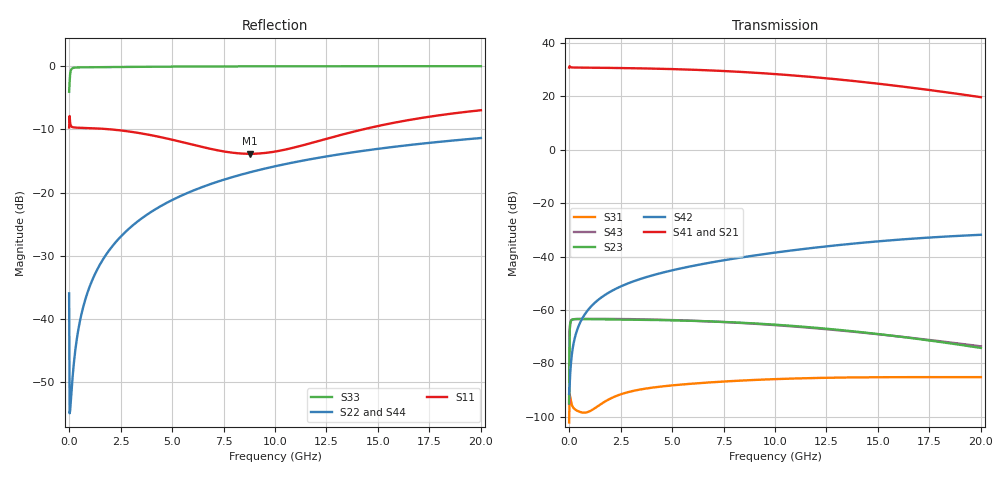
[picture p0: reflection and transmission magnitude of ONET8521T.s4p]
! *  ONET8521T
! * (C) Copyright 2011 Texas Instruments Incorporated. All rights reserved.
! ** This model is designed as an aid for customers of Texas Instruments.
! ** TI and its licensors and suppliers make no warranties, either expressed
! ** or implied, with respect to this model, including the warranties of
! ** merchantability or fitness for a particular purpose.  The model is
! ** provided solely on an "as is" basis.  The entire risk as to its quality
! ** and performance is with the customer.
! ** 1) THE ACCURACY OF THE MODELS PROVIDED TO YOUR COMPANY;
! ** 2) THE PROPER FUNCTIONING OF THESE MODELS IN YOUR DESIGN OR FOR ANY RESULTING
! ** APPLICATIONS; OR 3) INFRINGEMENT OF PATENTS, COPYRIGHTS OR INTELLECTUAL PROPERTY
! **  RIGHTS RESULTING FROM YOUR USE OF THESE HSPICE MODELS.
! ** TI PROVIDES MODELS AS A SERVICE TO OUR CUSTOMERS. YOU AND YOUR COMPANY
! ** SHALL NOT DISTRIBUTE, SELL OR GIVE THESE MODELS
! ** TO ANYONE ELSE WITHOUT PRIOR WRITTEN PERMISSION FROM TI.
! ** TI RESERVES THE RIGHT TO MAKE CHANGES TO OUR PRODUCTS OR TO DISCONTINUE
! ** ANY SEMICONDUCTOR PRODUCT OR SERVICE WITHOUT NOTICE, AND ADVISES OUR
! ** CUSTOMERS TO OBTAIN THE LATEST VERSION OF RELEVANT INFORMATION TO VERIFY,
! ** BEFORE PLACING ORDERS, THAT THE INFORMATION BEING RELIED ON IS CURRENT.
! ** PLEASE BE AWARE THAT YOUR RECEIPT AND USE OF THIS INFORMATION PROVIDED SHALL
! ** SERVE AS ACCEPTANCE OF THESE TERMS AND CONDITIONS. IF YOU DO NOT ACCEPT
! ** THESE TERMS, YOU SHOULD RETURN OR DESTROY THE MODELS AND ANY OTHER ACCOMPANYING
! ** INFORMATION IMMEDIATELY.
! *** ONET8521T ***
! *** 11.3 Gbps Limiting Transimpedance Amplifier with RSSI ***
! Touchstone Ver. 1.0
! Mon Jul  4 13:36:07 2011
! Number of ports is 4
! Port 1: In
! Port 2: Out+
! Port 3: Filter
! Port 4: Out-
# Hz	S	DB	R	50.000000
! SCATTERING PARAMETERS  :
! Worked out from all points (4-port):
!   802 points, 1 MHz to 20 GHz, reference 50 ohm
!   strongest paths, dB at 1 MHz, 4.995 GHz, 10.01 GHz, 15.01 GHz, 20 GHz:
!     S41: 30.8, 30.2, 28.3, 24.7, 19.7
!     S21: 30.8, 30.2, 28.3, 24.7, 19.6
!     S42: -91.4, -45.2, -38.5, -34.3, -31.8
!     S23: -95.0, -63.9, -65.5, -69.0, -74.2
!     S43: -95.0, -63.8, -65.7, -69.1, -73.6
!     S31: -102.1, -88.3, -85.9, -85.2, -85.1
!   lowest |S11| = -13.9 dB at 8.79 GHz (marker M1), VSWR 1.51, Z = 33.5 - j3.92 ohm
!   |S11| at or under -10 dB: 2.016 GHz to 14.28 GHz (12.26 GHz wide, 151 % of centre)
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1000000  -9.70 -172.3  -147.70 0.4  -123.32 117.9  -147.70 0.4
         30.78 2.8  -35.93 -83.9  -94.99 -61.3  -92.48 4.4
         -102.13 163.0  -183.67 -161.7  -4.05 -3.9  -183.67 -161.7
         30.78 -177.2  -91.45 4.1  -94.98 118.7  -35.93 -83.9
2.123241e9  -10.03 175.9  -121.18 81.3  -91.72 0.2  -121.18 81.4
            30.65 -33.2  -28.38 -92.8  -63.56 147.2  -52.79 84.8
            -92.76 -168.7  -118.30 85.2  -0.15 -177.8  -118.30 85.2
            30.64 146.8  -52.64 84.2  -63.35 -31.2  -28.39 -92.8
4.57006e9  -11.31 174.3  -113.85 63.9  -91.98 -0.8  -113.86 63.9
           30.30 -71.3  -21.92 -99.3  -63.81 108.4  -46.02 79.5
           -88.59 141.3  -111.86 78.7  -0.08 -178.6  -111.86 78.7
           30.30 108.9  -45.96 78.2  -63.67 -69.9  -21.92 -99.2
8.789574e9  -13.86 -163.9  -107.87 32.1  -92.50 2.4  -107.99 32.7
            28.94 -137.8  -16.78 -107.7  -64.95 41.5  -39.62 68.8
            -86.28 91.6  -106.84 69.3  -0.03 -179.1  -106.84 69.3
            28.95 42.5  -39.84 67.5  -65.06 -137.3  -16.76 -107.6
1.121143e10  -12.64 -145.5  -105.39 13.9  -92.49 5.8  -105.65 15.5
             27.61 -175.6  -15.03 -111.6  -66.18 3.9  -37.00 60.0
             -85.61 73.0  -105.20 65.1  -0.02 -179.3  -105.20 65.1
             27.63 4.7  -37.32 59.6  -66.37 -175.8  -15.00 -111.6
1.42325e10  -10.04 -137.3  -102.40 -8.5  -92.14 9.0  -102.87 -4.9
            25.38 138.7  -13.41 -115.7  -68.35 -41.4  -34.48 46.4
            -85.23 55.4  -103.74 60.9  -0.01 -179.5  -103.74 60.9
            25.41 -40.9  -34.83 47.5  -68.47 137.5  -13.39 -115.9
2e10  -6.97 -140.4  -96.41 -47.1  -91.32 10.7  -96.99 -40.0
      19.63 59.0  -11.37 -122.2  -74.21 -121.3  -31.80 17.1
      -85.15 33.9  -101.85 55.4  -0.01 -179.6  -101.85 55.4
      19.69 -120.1  -31.84 20.3  -73.61 57.5  -11.39 -122.4
